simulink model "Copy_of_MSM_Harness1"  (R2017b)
settings: Solver=FixedStepDiscrete  StartTime=0.0  StopTime=2  FixedStep=0.01  RelTol=1e-3  EnableMultiTasking=on
undefined symbols (not defined in the file): sigbuilder_block

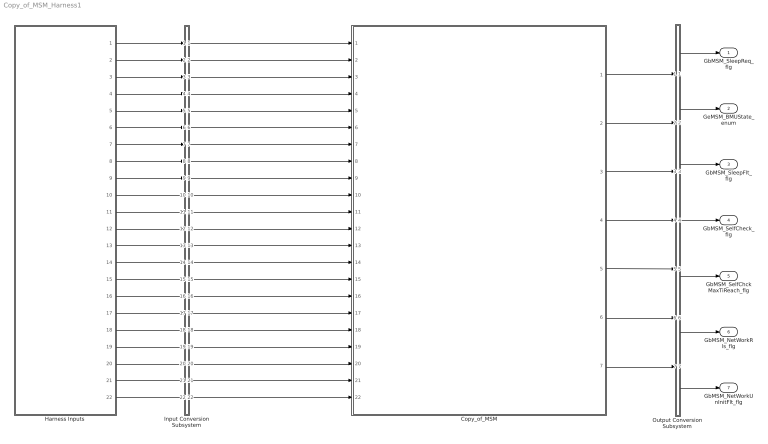
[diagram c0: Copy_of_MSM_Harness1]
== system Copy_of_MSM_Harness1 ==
  Copy_of_MSM : ModelReference  ModelNameDialog=Copy_of_MSM  SimulationMode=Normal  ModelReferenceVersion='M108C102'
  Harness Inputs : Subsystem  Tag=STV Subsys  LoadFcn=sigbuilder_block('load');  StartFcn=sigbuilder_block('start');  StopFcn=sigbuilder_block('stop');  ClipboardFcn=sigbuilder_block('clipboard');  mask(Sigbuilder block){tuvar=[0:10]}
      mask init:
      | if ~strcmp(get_param(bdroot(gcb),'SimulationStatus'),'stopped'),tuvar = sigbuilder_block('maskInit'); end
  Input Conversion Subsystem : Subsystem  Tag=__SLT_ICS__  Description=Signal spec. and routing
  Output Conversion Subsystem : Subsystem  Tag=__SLT_OCS__  Description=Signal spec. and routing
  GbMSM_SleepReq_flg : Outport  OutDataTypeStr=boolean  PortDimensions=[1]
  GeMSM_BMUState_enum : Outport  Port=2  OutDataTypeStr=uint8  PortDimensions=[1]
  GbMSM_SleepFlt_flg : Outport  Port=3  OutDataTypeStr=boolean  PortDimensions=[1]
  GbMSM_SelfCheck_flg : Outport  Port=4  OutDataTypeStr=boolean  PortDimensions=[1]
  GbMSM_SelfChckMaxTiReach_flg : Outport  Port=5  OutDataTypeStr=boolean  PortDimensions=[1]
  GbMSM_NetWorkRls_flg : Outport  Port=6  OutDataTypeStr=boolean  PortDimensions=[1]
  GbMSM_NetWorkUnInitFlt_flg : Outport  Port=7  OutDataTypeStr=boolean  PortDimensions=[1]
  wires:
  Harness Inputs/1(GbISP_SleepReqFbk_flg) -> Input Conversion Subsystem/1(Inport_1)
  Harness Inputs/2(GeISP_BsicSysMod_enum) -> Input Conversion Subsystem/2(Inport_2)
  Harness Inputs/3(GbHVL_HvilSelfCheck_flg) -> Input Conversion Subsystem/3(Inport_3)
  Harness Inputs/4(GbCDP_CellVoltSelfChck_flg) -> Input Conversion Subsystem/4(Inport_4)
  Harness Inputs/5(GbCDP_CellTempSelfChck_flg) -> Input Conversion Subsystem/5(Inport_5)
  Harness Inputs/6(GbHDP_PackCrntSelfChck_flg) -> Input Conversion Subsystem/6(Inport_6)
  Harness Inputs/7(GbHDP_PackVoltSelfChck_flg) -> Input Conversion Subsystem/7(Inport_7)
  Harness Inputs/8(GbISO_ResSelfCheck_flg) -> Input Conversion Subsystem/8(Inport_8)
  Harness Inputs/9(GbCSH_CrashFlt_flg) -> Input Conversion Subsystem/9(Inport_9)
  Harness Inputs/10(GbBPM_BMUSpyNormal_flg) -> Input Conversion Subsystem/10(Inport_10)
  Harness Inputs/11(GeFTC_FltLevel_enum) -> Input Conversion Subsystem/11(Inport_11)
  Harness Inputs/12(GeVDP_DriveRqst_enum) -> Input Conversion Subsystem/12(Inport_12)
  Harness Inputs/13(GcWSM_WakeupSrc_numb) -> Input Conversion Subsystem/13(Inport_13)
  Harness Inputs/14(GeCTC_CtrCtlState_enum) -> Input Conversion Subsystem/14(Inport_14)
  Harness Inputs/15(GeISP_NetWkUpSt_enum) -> Input Conversion Subsystem/15(Inport_15)
  Harness Inputs/16(GbWSM_Kl15WkUpPrs_flg) -> Input Conversion Subsystem/16(Inport_16)
  Harness Inputs/17(GbWSM_ACWkUpPrs_flg) -> Input Conversion Subsystem/17(Inport_17)
  Harness Inputs/18(GbWSM_DCWkUpPrs_flg) -> Input Conversion Subsystem/18(Inport_18)
  Harness Inputs/19(GbWSM_EDCWkUpPrs_flg) -> Input Conversion Subsystem/19(Inport_19)
  Harness Inputs/20(GbWSM_TplWkUpPrs_flg) -> Input Conversion Subsystem/20(Inport_20)
  Harness Inputs/21(GbISP_TFThmRnwyfDet_flg) -> Input Conversion Subsystem/21(Inport_21)
  Harness Inputs/22(GbWSM_CANWkUpPrs_flg) -> Input Conversion Subsystem/22(Inport_22)
  Output Conversion Subsystem/1(Outport_1) -> GbMSM_SleepReq_flg/1
  Output Conversion Subsystem/2(Outport_2) -> GeMSM_BMUState_enum/1
  Output Conversion Subsystem/3(Outport_3) -> GbMSM_SleepFlt_flg/1
  Output Conversion Subsystem/4(Outport_4) -> GbMSM_SelfCheck_flg/1
  Output Conversion Subsystem/5(Outport_5) -> GbMSM_SelfChckMaxTiReach_flg/1
  Output Conversion Subsystem/6(Outport_6) -> GbMSM_NetWorkRls_flg/1
  Output Conversion Subsystem/7(Outport_7) -> GbMSM_NetWorkUnInitFlt_flg/1
  Input Conversion Subsystem/1(Outport_1) -> Copy_of_MSM/1
  Input Conversion Subsystem/2(Outport_2) -> Copy_of_MSM/2
  Input Conversion Subsystem/3(Outport_3) -> Copy_of_MSM/3
  Input Conversion Subsystem/4(Outport_4) -> Copy_of_MSM/4
  Input Conversion Subsystem/5(Outport_5) -> Copy_of_MSM/5
  Input Conversion Subsystem/6(Outport_6) -> Copy_of_MSM/6
  Input Conversion Subsystem/7(Outport_7) -> Copy_of_MSM/7
  Input Conversion Subsystem/8(Outport_8) -> Copy_of_MSM/8
  Input Conversion Subsystem/9(Outport_9) -> Copy_of_MSM/9
  Input Conversion Subsystem/10(Outport_10) -> Copy_of_MSM/10
  Input Conversion Subsystem/11(Outport_11) -> Copy_of_MSM/11
  Input Conversion Subsystem/12(Outport_12) -> Copy_of_MSM/12
  Input Conversion Subsystem/13(Outport_13) -> Copy_of_MSM/13
  Input Conversion Subsystem/14(Outport_14) -> Copy_of_MSM/14
  Input Conversion Subsystem/15(Outport_15) -> Copy_of_MSM/15
  Input Conversion Subsystem/16(Outport_16) -> Copy_of_MSM/16
  Input Conversion Subsystem/17(Outport_17) -> Copy_of_MSM/17
  Input Conversion Subsystem/18(Outport_18) -> Copy_of_MSM/18
  Input Conversion Subsystem/19(Outport_19) -> Copy_of_MSM/19
  Input Conversion Subsystem/20(Outport_20) -> Copy_of_MSM/20
  Input Conversion Subsystem/21(Outport_21) -> Copy_of_MSM/21
  Input Conversion Subsystem/22(Outport_22) -> Copy_of_MSM/22
  Copy_of_MSM/1 -> Output Conversion Subsystem/1(Inport_1)
  Copy_of_MSM/2 -> Output Conversion Subsystem/2(Inport_2)
  Copy_of_MSM/3 -> Output Conversion Subsystem/3(Inport_3)
  Copy_of_MSM/4 -> Output Conversion Subsystem/4(Inport_4)
  Copy_of_MSM/5 -> Output Conversion Subsystem/5(Inport_5)
  Copy_of_MSM/6 -> Output Conversion Subsystem/6(Inport_6)
  Copy_of_MSM/7 -> Output Conversion Subsystem/7(Inport_7)

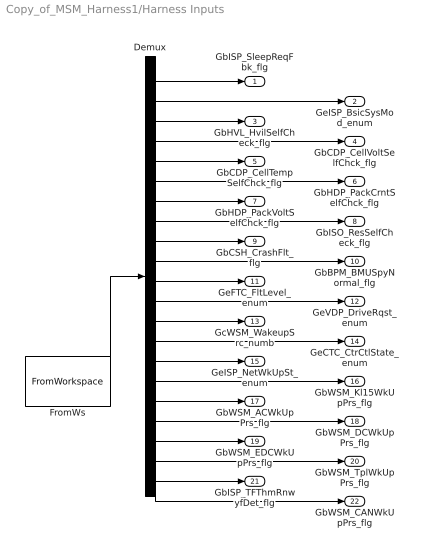
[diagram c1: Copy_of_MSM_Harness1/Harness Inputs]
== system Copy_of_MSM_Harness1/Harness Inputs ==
  Demux : Demux  Tag=STV Demux  Outputs=22
  FromWs : FromWorkspace  Tag=STV FromWs  VariableName=tuvar  SampleTime=0
  GbISP_SleepReqFbk_flg : Outport  Tag=STV Outport
  GeISP_BsicSysMod_enum : Outport  Tag=STV Outport  Port=2
  GbHVL_HvilSelfCheck_flg : Outport  Tag=STV Outport  Port=3
  GbCDP_CellVoltSelfChck_flg : Outport  Tag=STV Outport  Port=4
  GbCDP_CellTempSelfChck_flg : Outport  Tag=STV Outport  Port=5
  GbHDP_PackCrntSelfChck_flg : Outport  Tag=STV Outport  Port=6
  GbHDP_PackVoltSelfChck_flg : Outport  Tag=STV Outport  Port=7
  GbISO_ResSelfCheck_flg : Outport  Tag=STV Outport  Port=8
  GbCSH_CrashFlt_flg : Outport  Tag=STV Outport  Port=9
  GbBPM_BMUSpyNormal_flg : Outport  Tag=STV Outport  Port=10
  GeFTC_FltLevel_enum : Outport  Tag=STV Outport  Port=11
  GeVDP_DriveRqst_enum : Outport  Tag=STV Outport  Port=12
  GcWSM_WakeupSrc_numb : Outport  Tag=STV Outport  Port=13
  GeCTC_CtrCtlState_enum : Outport  Tag=STV Outport  Port=14
  GeISP_NetWkUpSt_enum : Outport  Tag=STV Outport  Port=15
  GbWSM_Kl15WkUpPrs_flg : Outport  Tag=STV Outport  Port=16
  GbWSM_ACWkUpPrs_flg : Outport  Tag=STV Outport  Port=17
  GbWSM_DCWkUpPrs_flg : Outport  Tag=STV Outport  Port=18
  GbWSM_EDCWkUpPrs_flg : Outport  Tag=STV Outport  Port=19
  GbWSM_TplWkUpPrs_flg : Outport  Tag=STV Outport  Port=20
  GbISP_TFThmRnwyfDet_flg : Outport  Tag=STV Outport  Port=21
  GbWSM_CANWkUpPrs_flg : Outport  Tag=STV Outport  Port=22
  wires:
  FromWs/1 -> Demux/1
  Demux/1 -> GbISP_SleepReqFbk_flg/1
  Demux/2 -> GeISP_BsicSysMod_enum/1
  Demux/3 -> GbHVL_HvilSelfCheck_flg/1
  Demux/4 -> GbCDP_CellVoltSelfChck_flg/1
  Demux/5 -> GbCDP_CellTempSelfChck_flg/1
  Demux/6 -> GbHDP_PackCrntSelfChck_flg/1
  Demux/7 -> GbHDP_PackVoltSelfChck_flg/1
  Demux/8 -> GbISO_ResSelfCheck_flg/1
  Demux/9 -> GbCSH_CrashFlt_flg/1
  Demux/10 -> GbBPM_BMUSpyNormal_flg/1
  Demux/11 -> GeFTC_FltLevel_enum/1
  Demux/12 -> GeVDP_DriveRqst_enum/1
  Demux/13 -> GcWSM_WakeupSrc_numb/1
  Demux/14 -> GeCTC_CtrCtlState_enum/1
  Demux/15 -> GeISP_NetWkUpSt_enum/1
  Demux/16 -> GbWSM_Kl15WkUpPrs_flg/1
  Demux/17 -> GbWSM_ACWkUpPrs_flg/1
  Demux/18 -> GbWSM_DCWkUpPrs_flg/1
  Demux/19 -> GbWSM_EDCWkUpPrs_flg/1
  Demux/20 -> GbWSM_TplWkUpPrs_flg/1
  Demux/21 -> GbISP_TFThmRnwyfDet_flg/1
  Demux/22 -> GbWSM_CANWkUpPrs_flg/1

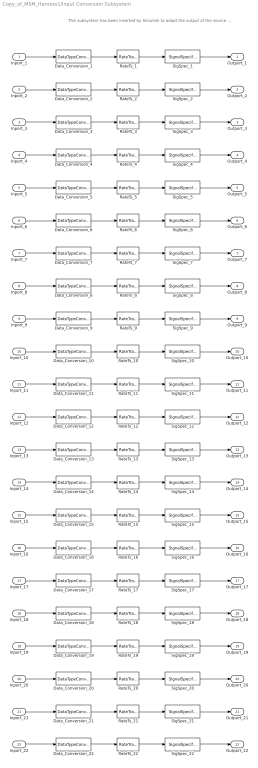
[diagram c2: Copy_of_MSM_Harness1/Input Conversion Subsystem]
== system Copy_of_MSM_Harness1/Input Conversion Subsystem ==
  note: This subsystem has been inserted by Simulink to adapt the output of the source blocks to the interface required by the harnessed component. Modifying the contents of this subsystem may result in compilation and simulation failure.
  Inport_1 : Inport
  Inport_2 : Inport  Port=2
  Inport_3 : Inport  Port=3
  Inport_4 : Inport  Port=4
  Inport_5 : Inport  Port=5
  Inport_6 : Inport  Port=6
  Inport_7 : Inport  Port=7
  Inport_8 : Inport  Port=8
  Inport_9 : Inport  Port=9
  Inport_10 : Inport  Port=10
  Inport_11 : Inport  Port=11
  Inport_12 : Inport  Port=12
  Inport_13 : Inport  Port=13
  Inport_14 : Inport  Port=14
  Inport_15 : Inport  Port=15
  Inport_16 : Inport  Port=16
  Inport_17 : Inport  Port=17
  Inport_18 : Inport  Port=18
  Inport_19 : Inport  Port=19
  Inport_20 : Inport  Port=20
  Inport_21 : Inport  Port=21
  Inport_22 : Inport  Port=22
  Data_Conversion_{1,3..10,16..22} (16 alike) : DataTypeConversion  OutDataTypeStr=boolean
  Data_Conversion_{2,11..12,14..15} (5 alike) : DataTypeConversion  OutDataTypeStr=uint8
  Data_Conversion_13 : DataTypeConversion  OutDataTypeStr=uint16
  RateTs_{1..22} (22 alike) : RateTransition  OutPortSampleTime=0.01
  SigSpec_{1,3..9,21} (9 alike) : SignalSpecification  OutDataTypeStr=boolean  Unit=flag  Dimensions=[1]  SampleTime=0.01
  SigSpec_{10,16..20,22} (7 alike) : SignalSpecification  OutDataTypeStr=boolean  Unit=flg  Dimensions=[1]  SampleTime=0.01
  SigSpec_{2,11..12,14..15} (5 alike) : SignalSpecification  OutDataTypeStr=uint8  Unit=enum  Dimensions=[1]  SampleTime=0.01
  SigSpec_13 : SignalSpecification  OutDataTypeStr=uint16  Unit=numb  Dimensions=[1]  SampleTime=0.01
  Outport_1 : Outport
  Outport_2 : Outport  Port=2
  Outport_3 : Outport  Port=3
  Outport_4 : Outport  Port=4
  Outport_5 : Outport  Port=5
  Outport_6 : Outport  Port=6
  Outport_7 : Outport  Port=7
  Outport_8 : Outport  Port=8
  Outport_9 : Outport  Port=9
  Outport_10 : Outport  Port=10
  Outport_11 : Outport  Port=11
  Outport_12 : Outport  Port=12
  Outport_13 : Outport  Port=13
  Outport_14 : Outport  Port=14
  Outport_15 : Outport  Port=15
  Outport_16 : Outport  Port=16
  Outport_17 : Outport  Port=17
  Outport_18 : Outport  Port=18
  Outport_19 : Outport  Port=19
  Outport_20 : Outport  Port=20
  Outport_21 : Outport  Port=21
  Outport_22 : Outport  Port=22
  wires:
  SigSpec_1/1 -> Outport_1/1
  RateTs_1/1 -> SigSpec_1/1
  Data_Conversion_1/1 -> RateTs_1/1
  Inport_1/1 -> Data_Conversion_1/1
  SigSpec_2/1 -> Outport_2/1
  RateTs_2/1 -> SigSpec_2/1
  Data_Conversion_2/1 -> RateTs_2/1
  Inport_2/1 -> Data_Conversion_2/1
  SigSpec_3/1 -> Outport_3/1
  RateTs_3/1 -> SigSpec_3/1
  Data_Conversion_3/1 -> RateTs_3/1
  Inport_3/1 -> Data_Conversion_3/1
  SigSpec_4/1 -> Outport_4/1
  RateTs_4/1 -> SigSpec_4/1
  Data_Conversion_4/1 -> RateTs_4/1
  Inport_4/1 -> Data_Conversion_4/1
  SigSpec_5/1 -> Outport_5/1
  RateTs_5/1 -> SigSpec_5/1
  Data_Conversion_5/1 -> RateTs_5/1
  Inport_5/1 -> Data_Conversion_5/1
  SigSpec_6/1 -> Outport_6/1
  RateTs_6/1 -> SigSpec_6/1
  Data_Conversion_6/1 -> RateTs_6/1
  Inport_6/1 -> Data_Conversion_6/1
  SigSpec_7/1 -> Outport_7/1
  RateTs_7/1 -> SigSpec_7/1
  Data_Conversion_7/1 -> RateTs_7/1
  Inport_7/1 -> Data_Conversion_7/1
  SigSpec_8/1 -> Outport_8/1
  RateTs_8/1 -> SigSpec_8/1
  Data_Conversion_8/1 -> RateTs_8/1
  Inport_8/1 -> Data_Conversion_8/1
  SigSpec_9/1 -> Outport_9/1
  RateTs_9/1 -> SigSpec_9/1
  Data_Conversion_9/1 -> RateTs_9/1
  Inport_9/1 -> Data_Conversion_9/1
  SigSpec_10/1 -> Outport_10/1
  RateTs_10/1 -> SigSpec_10/1
  Data_Conversion_10/1 -> RateTs_10/1
  Inport_10/1 -> Data_Conversion_10/1
  SigSpec_11/1 -> Outport_11/1
  RateTs_11/1 -> SigSpec_11/1
  Data_Conversion_11/1 -> RateTs_11/1
  Inport_11/1 -> Data_Conversion_11/1
  SigSpec_12/1 -> Outport_12/1
  RateTs_12/1 -> SigSpec_12/1
  Data_Conversion_12/1 -> RateTs_12/1
  Inport_12/1 -> Data_Conversion_12/1
  SigSpec_13/1 -> Outport_13/1
  RateTs_13/1 -> SigSpec_13/1
  Data_Conversion_13/1 -> RateTs_13/1
  Inport_13/1 -> Data_Conversion_13/1
  SigSpec_14/1 -> Outport_14/1
  RateTs_14/1 -> SigSpec_14/1
  Data_Conversion_14/1 -> RateTs_14/1
  Inport_14/1 -> Data_Conversion_14/1
  SigSpec_15/1 -> Outport_15/1
  RateTs_15/1 -> SigSpec_15/1
  Data_Conversion_15/1 -> RateTs_15/1
  Inport_15/1 -> Data_Conversion_15/1
  SigSpec_16/1 -> Outport_16/1
  RateTs_16/1 -> SigSpec_16/1
  Data_Conversion_16/1 -> RateTs_16/1
  Inport_16/1 -> Data_Conversion_16/1
  SigSpec_17/1 -> Outport_17/1
  RateTs_17/1 -> SigSpec_17/1
  Data_Conversion_17/1 -> RateTs_17/1
  Inport_17/1 -> Data_Conversion_17/1
  SigSpec_18/1 -> Outport_18/1
  RateTs_18/1 -> SigSpec_18/1
  Data_Conversion_18/1 -> RateTs_18/1
  Inport_18/1 -> Data_Conversion_18/1
  SigSpec_19/1 -> Outport_19/1
  RateTs_19/1 -> SigSpec_19/1
  Data_Conversion_19/1 -> RateTs_19/1
  Inport_19/1 -> Data_Conversion_19/1
  SigSpec_20/1 -> Outport_20/1
  RateTs_20/1 -> SigSpec_20/1
  Data_Conversion_20/1 -> RateTs_20/1
  Inport_20/1 -> Data_Conversion_20/1
  SigSpec_21/1 -> Outport_21/1
  RateTs_21/1 -> SigSpec_21/1
  Data_Conversion_21/1 -> RateTs_21/1
  Inport_21/1 -> Data_Conversion_21/1
  SigSpec_22/1 -> Outport_22/1
  RateTs_22/1 -> SigSpec_22/1
  Data_Conversion_22/1 -> RateTs_22/1
  Inport_22/1 -> Data_Conversion_22/1

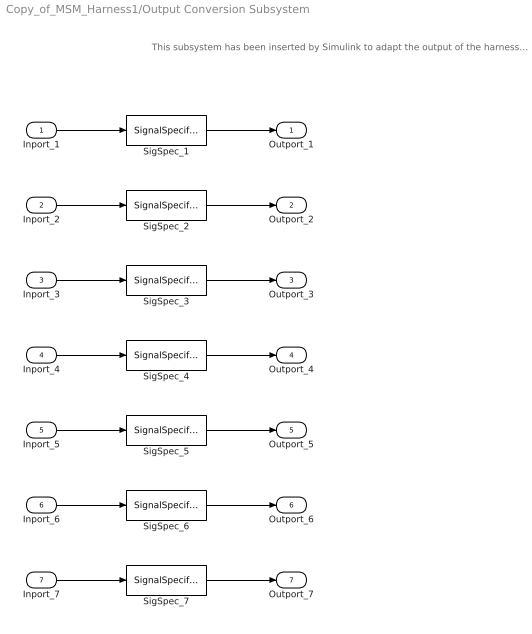
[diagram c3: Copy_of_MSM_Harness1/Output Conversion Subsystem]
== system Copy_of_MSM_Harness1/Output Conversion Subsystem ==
  note: This subsystem has been inserted by Simulink to adapt the output of the harnessed component to the interface required by the sink blocks. Modifying the contents of this subsystem may result in compilation and simulation failure.
  Inport_1 : Inport
  Inport_2 : Inport  Port=2
  Inport_3 : Inport  Port=3
  Inport_4 : Inport  Port=4
  Inport_5 : Inport  Port=5
  Inport_6 : Inport  Port=6
  Inport_7 : Inport  Port=7
  SigSpec_1 : SignalSpecification  OutDataTypeStr=boolean  Unit=flg  Dimensions=[1]  SampleTime=0.01
  SigSpec_2 : SignalSpecification  OutDataTypeStr=uint8  Unit=enum  Dimensions=[1]  SampleTime=0.01
  SigSpec_{3..7} (5 alike) : SignalSpecification  OutDataTypeStr=boolean  Unit=flag  Dimensions=[1]  SampleTime=0.01
  Outport_1 : Outport
  Outport_2 : Outport  Port=2
  Outport_3 : Outport  Port=3
  Outport_4 : Outport  Port=4
  Outport_5 : Outport  Port=5
  Outport_6 : Outport  Port=6
  Outport_7 : Outport  Port=7
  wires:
  Inport_1/1 -> SigSpec_1/1
  SigSpec_1/1 -> Outport_1/1
  Inport_2/1 -> SigSpec_2/1
  SigSpec_2/1 -> Outport_2/1
  Inport_3/1 -> SigSpec_3/1
  SigSpec_3/1 -> Outport_3/1
  Inport_4/1 -> SigSpec_4/1
  SigSpec_4/1 -> Outport_4/1
  Inport_5/1 -> SigSpec_5/1
  SigSpec_5/1 -> Outport_5/1
  Inport_6/1 -> SigSpec_6/1
  SigSpec_6/1 -> Outport_6/1
  Inport_7/1 -> SigSpec_7/1
  SigSpec_7/1 -> Outport_7/1
